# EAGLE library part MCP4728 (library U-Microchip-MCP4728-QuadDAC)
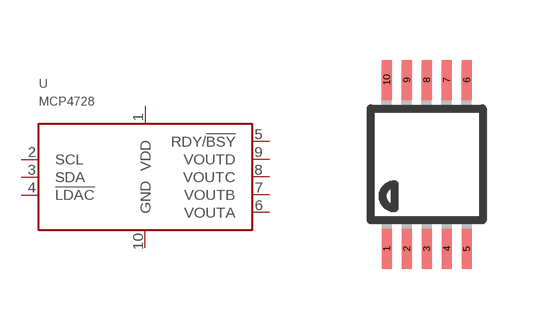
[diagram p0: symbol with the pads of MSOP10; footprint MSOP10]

Designator prefix -

## MCP4728  [MSOP10]
1  VDD
2  SCL
3  SDA
4  !LDAC
5  RDY/!BSY
6  VOUTA
7  VOUTB
8  VOUTC
9  VOUTD
10  GND

## Footprint MSOP10 (pad centres in mm)
10-Lead Mini Small Outline Package [MSOP] (RM-10) Source: http://www.analog.com/UploadedFiles/Data_Sheets/35641221898805SSM2167_b.pdf COMPLIANT TO JEDEC STANDARDS MO-187BA
smd 0.25 x 1: 1 -1,-2.113; 2 -0.5,-2.113; 3 0,-2.113; 4 0.5,-2.113; 5 1,-2.113; 6 1,2.113; 7 0.5,2.113; 8 0,2.113; 9 -0.5,2.113; 10 -1,2.113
